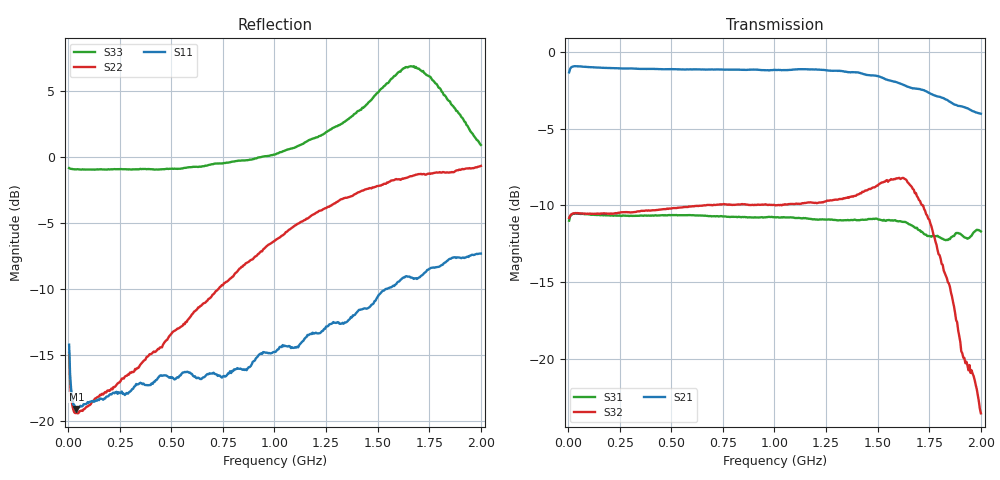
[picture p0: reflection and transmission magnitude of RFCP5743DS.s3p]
!Agilent Technologies,E5071C,MY46521875,B.13.32
!Date: Tue Aug 25 13:44:17 2026
!Data & Calibration Information:
!Freq	S11:SOLT3(ON)	S12:SOLT3(ON)	S13:SOLT3(ON)
!	S21:SOLT3(ON)	S22:SOLT3(ON)	S23:SOLT3(ON)
!	S31:SOLT3(ON)	S32:SOLT3(ON)	S33:SOLT3(ON)
!PortZ  Port1:75+j0  Port2:75+j0  Port3:75+j0
!Above PortZ is port z conversion or system Z0 setting when saving the data.
!When reading, reference impedance value at option line is always used.
# Hz S RI R 75
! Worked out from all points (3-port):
!   400 points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, 5.1 MHz to 2 GHz, reference 75 ohm
!   strongest paths, dB at 5.1 MHz, 505.1 MHz, 1.005 GHz, 1.505 GHz, 2 GHz:
!     S21: -1.3, -1.1, -1.2, -1.6, -4.0
!     S32: -10.8, -10.2, -10.0, -8.6, -23.6
!     S31: -11.0, -10.6, -10.8, -10.9, -11.7
!   lowest |S11| = -19.1 dB at 40.1 MHz (marker M1), VSWR 1.25, Z = 60.1 + j0.768 ohm
!   |S11| at or under -10 dB: start of sweep to 1.546 GHz
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5099750  -0.1602 0.1098  0.8586 0.1061  -0.2826 -0.0349
         0.8505 0.1088  -0.1479 0.1048  -0.2803 -0.0351
         -0.2792 -0.0361  -0.2852 -0.0336  -0.9086 0.0122
4.0098e7  -0.1106 0.00632  0.9052 0.00133  -0.2976 0.00534
          0.8982 -0.00349  -0.1061 0.0149  -0.2958 0.00876
          -0.2966 0.00349  -0.2978 0.00667  -0.8981 0.0216
1.00505e9  -0.1616 -0.0844  0.7554 -0.3594  -0.2517 0.2009
           0.7722 -0.4068  -0.341 0.3433  -0.2188 0.2424
           -0.2185 0.1889  -0.1916 0.2511  -0.9318 0.4253
1.470026e9  -0.2472 -0.1212  0.6009 -0.3923  -0.2949 0.3555
            0.5859 -0.5988  -0.4325 0.6258  -0.2453 0.418
            -0.1546 0.2394  -0.2492 0.2578  -1.635 0.2199
1.565022e9  -0.2885 -0.1403  0.5809 -0.3727  -0.3535 0.3583
            0.5194 -0.6148  -0.4448 0.6827  -0.3028 0.4517
            -0.1414 0.2437  -0.315 0.2207  -1.967 -0.2189
1.625019e9  -0.3159 -0.1499  0.5653 -0.3578  -0.405 0.3122
            0.4735 -0.6203  -0.4506 0.694  -0.3738 0.4257
            -0.1355 0.2437  -0.3556 0.1553  -2.036 -0.7578
1.700015e9  -0.3208 -0.1379  0.5418 -0.3803  -0.4185 0.2043
            0.4258 -0.6256  -0.4765 0.7186  -0.429 0.3178
            -0.1178 0.2342  -0.3254 0.0474  -1.599 -1.461
1.770012e9  -0.3607 -0.1239  0.5534 -0.3957  -0.3685 0.0936
            0.3902 -0.609  -0.483 0.7236  -0.4007 0.2092
            -0.0975 0.2317  -0.2536 0.00596  -0.9421 -1.705
1.870006e9  -0.4037 -0.1031  0.5648 -0.4094  -0.2607 0.0221
            0.3401 -0.5822  -0.478 0.7359  -0.3044 0.1107
            -0.0686 0.2413  -0.1473 0.00955  -0.2051 -1.528
2e9  -0.4258 -0.0634  0.5686 -0.4266  -0.1657 0.0133
     0.2964 -0.5542  -0.473 0.7956  -0.1926 0.0829
     -0.044 0.256  -0.0293 0.0594  0.2296 -1.088
